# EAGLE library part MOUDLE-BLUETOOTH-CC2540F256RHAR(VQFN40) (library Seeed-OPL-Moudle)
317070005
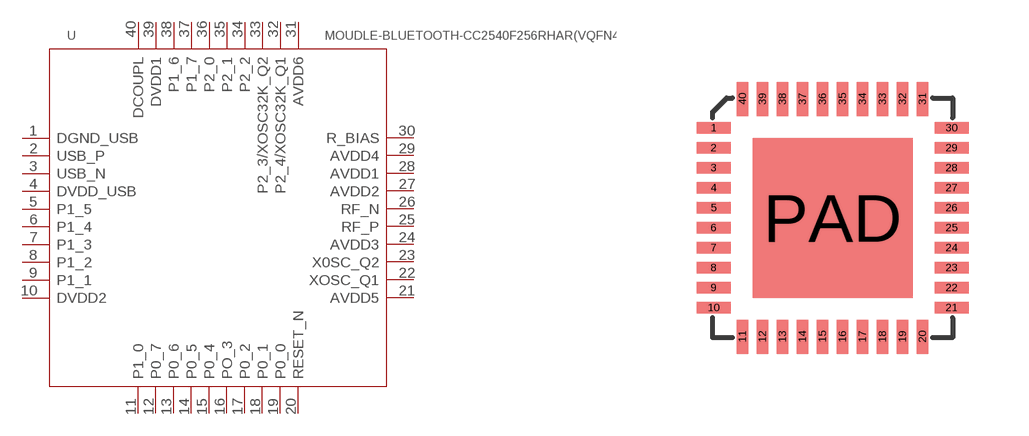
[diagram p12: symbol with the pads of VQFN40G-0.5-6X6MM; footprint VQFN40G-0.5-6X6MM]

Designator prefix U

## MOUDLE-BLUETOOTH-CC2540F256RHAR(VQFN40) (MPN: CC2540F256RHAR; VALUE: CC2540F256RHAR)  [VQFN40G-0.5-6X6MM]
1  DGND_USB
2  USB_P
3  USB_N
4  DVDD_USB
5  P1_5
6  P1_4
7  P1_3
8  P1_2
9  P1_1
10  DVDD2
11  P1_0
12  P0_7
13  P0_6
14  P0_5
15  P0_4
16  PO_3
17  P0_2
18  P0_1
19  P0_0
20  RESET_N
21  AVDD5
22  XOSC_Q1
23  X0SC_Q2
24  AVDD3
25  RF_P
26  RF_N
27  AVDD2
28  AVDD1
29  AVDD4
30  R_BIAS
31  AVDD6
32  P2_4/XOSC32K_Q1
33  P2_3/XOSC32K_Q2
34  P2_2
35  P2_1
36  P2_0
37  P1_7
38  P1_6
39  DVDD1
40  DCOUPL

## Footprint VQFN40G-0.5-6X6MM (pad centres in mm)
smd 0.85 x 0.28: 1 -2.975,2.25; 2 -2.975,1.75; 3 -2.975,1.25; 4 -2.975,0.75; 5 -2.975,0.25; 6 -2.975,-0.25; 7 -2.975,-0.75; 8 -2.975,-1.25; 9 -2.975,-1.75; 10 -2.975,-2.25; 21 2.975,-2.25; 22 2.975,-1.75; 23 2.975,-1.25; 24 2.975,-0.75; 25 2.975,-0.25; 26 2.975,0.25; 27 2.975,0.75; 28 2.975,1.25; 29 2.975,1.75; 30 2.975,2.25
smd 0.28 x 0.85: 11 -2.25,-2.975; 12 -1.75,-2.975; 13 -1.25,-2.975; 14 -0.75,-2.975; 15 -0.25,-2.975; 16 0.25,-2.975; 17 0.75,-2.975; 18 1.25,-2.975; 19 1.75,-2.975; 20 2.25,-2.975; 31 2.25,2.975; 32 1.75,2.975; 33 1.25,2.975; 34 0.75,2.975; 35 0.25,2.975; 36 -0.25,2.975; 37 -0.75,2.975; 38 -1.25,2.975; 39 -1.75,2.975; 40 -2.25,2.975
smd 4 x 4: PAD 0,0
